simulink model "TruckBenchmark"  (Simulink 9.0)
settings: Solver=ode23s  StartTime=0.0  StopTime=inf  FixedStep=0.1  MaxStep=1  RelTol=1e-3  EnableMultiTasking=on
StartFcn:
  | tic
StopFcn:
  | simt=toc;
  | fprintf('Simulation time %.3f s
  | ',simt)
  | TruckBenchmark_Evaluation
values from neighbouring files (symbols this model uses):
  road = scenario.road    [runSim.m]
undefined symbols (not defined in the file or in its folder): A_egrmax, A_vgtmax, AFs, Area, BSR_opt, C_d, c_egr, c_f1, c_f2, c_fricVec, c_mlin, c_mVec, c_pa, c_pe, c_phi2, c_pi, c_psi2, c_r0, c_r1, c_va, c_vgt1, c_vgt2, c_volVec, c_wphiVec, c_wpsiVec, d_pipe, eta_cmax, eta_igch, eta_sc, eta_tmmax, g, gamma_a, gamma_c, gamma_e, h_tot, J_t, K_t, l_pipe, limit_m_f, limit_n_e, m, model, n_cyl, n_pipe, omega_t_Init, p_amb, p_em_Init, p_im_Init, pi_copt, PI_egropt, Q_c, q_HV, R_a, r_c, R_c, R_e, R_t, rho, scenario, T_1_Init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
libraries: controller x1, simulink x1

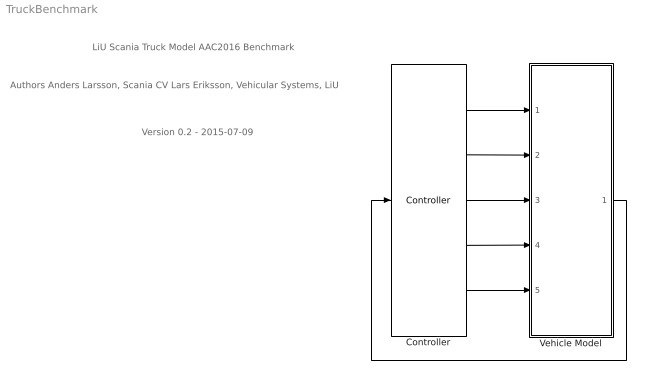
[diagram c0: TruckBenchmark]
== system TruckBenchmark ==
  note: Version 0.2 - 2015-07-09
  note: Authors Anders Larsson, Scania CV Lars Eriksson, Vehicular Systems, LiU
  note: LiU Scania Truck Model AAC2016 Benchmark
  Controller : controller/Controller
  Vehicle Model : Subsystem
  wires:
  Vehicle Model/1(Sensor Buss) -> Controller/1
  Controller/1 -> Vehicle Model/1(gear)
  Controller/2 -> Vehicle Model/2(u_vgt)
  Controller/3 -> Vehicle Model/3(u_egr)
  Controller/4 -> Vehicle Model/4(u_delta)
  Controller/5 -> Vehicle Model/5(F_brake)

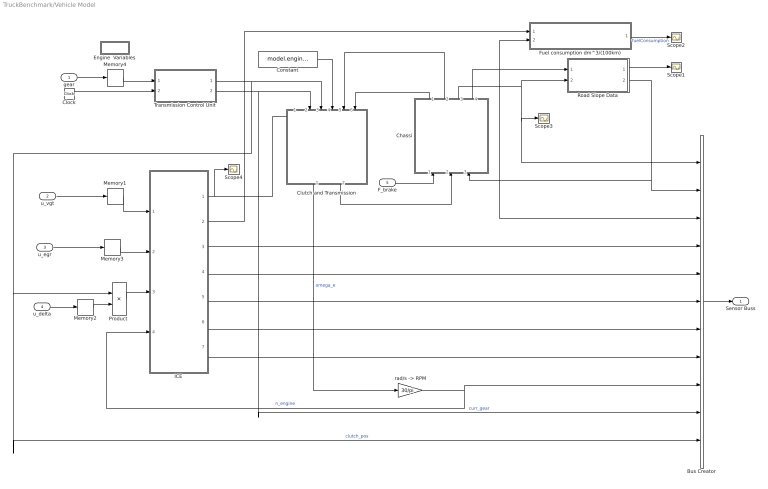
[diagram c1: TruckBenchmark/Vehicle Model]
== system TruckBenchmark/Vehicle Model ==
  gear : Inport
  u_vgt : Inport  Port=2
  u_egr : Inport  Port=3
  u_delta : Inport  Port=4
  F_brake : Inport  Port=5
  Bus Creator : BusCreator  Inputs=11
  Chassi : Subsystem
  Clock : Clock
  Clutch and Transmission : Subsystem
  Constant : Constant  Value=model.engine.J_e
  Engine  Variables : Subsystem
  Fuel consumption dm^3/(100km) : MATLAB Function  TreatAsAtomicUnit=on
  ICE : Subsystem
  Memory1 : Memory  InitialCondition=40
  Memory2 : Memory
  Memory3 : Memory
  Memory4 : Memory  InitialCondition=scenario.gear_init
  "Product " : Product  Inputs=**
  Road Slope Data : Subsystem
  Scope{1..4} (4 alike) : Scope
  Transmission Control Unit : MATLAB Function  TreatAsAtomicUnit=on
  "rad/s -> RPM" : Gain  Gain=30/pi
  Sensor Buss : Outport
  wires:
  ICE/1(M_e) -> Clutch and Transmission/1(M_e [Nm]), Scope4/1
  Road Slope Data/2(slope [rad]) -> Chassi/3(Slope), Bus Creator/2
  Chassi/3(Vehicle Speed[km/h]) -> Road Slope Data/2(v [km/h]), Bus Creator/1, Scope3/1
  ICE/2(m_fuelTot) -> Fuel consumption dm^3/(100km)/1(m_fuelTot)
  Fuel consumption dm^3/(100km)/1(fuelConsumption) -> Scope2/1  "fuelConsumption"
  Chassi/4(Distance [m]) -> Road Slope Data/1(x_distance), Fuel consumption dm^3/(100km)/2(x_distance), Bus Creator/3
  ICE/3(r_lambdaOut) -> Bus Creator/4
  ICE/4(p_inletManifold) -> Bus Creator/5
  ICE/5(r_egr) -> Bus Creator/6
  ICE/6(W_c) -> Bus Creator/7
  u_vgt/1 -> Memory1/1
  u_egr/1 -> Memory3/1
  Memory3/1 -> ICE/2(u_egr)
  F_brake/1 -> Chassi/1(Brake Pedal [%])
  Bus Creator/1 -> Sensor Buss/1
  Clutch and Transmission/2(w_wheel [rad/s]) -> Chassi/2(Wheel speed [rad/s])
  Clutch and Transmission/1(w_e [rad/s]) -> "rad/s -> RPM"/1  "omega_e"
  Chassi/1(Vehicle Inertia [kgm^2]) -> Clutch and Transmission/6(J_veh)
  Chassi/2(Vehicle Torque [Nm]) -> Clutch and Transmission/5(M_veh [Nm])
  "rad/s -> RPM"/1 -> ICE/4(n_e), Bus Creator/9  "n_engine"
  Constant/1 -> Clutch and Transmission/4(J_e)
  Memory1/1 -> ICE/1(u_vgt)
  Transmission Control Unit/2(gear_out) -> Bus Creator/10, Clutch and Transmission/2(Gear)  "curr_gear"
  Clock/1 -> Transmission Control Unit/2(time)
  gear/1 -> Memory4/1
  "Product "/1 -> ICE/3(u_delta)
  Transmission Control Unit/1(clutch) -> Clutch and Transmission/3(Clutch Pos [0...1]), "Product "/1, Bus Creator/11  "clutch_pos"
  u_delta/1 -> Memory2/1
  Memory4/1 -> Transmission Control Unit/1(gear_ref)
  ICE/7(n_t) -> Bus Creator/8
  Road Slope Data/1(altitude [m]) -> Scope1/1
  Memory2/1 -> "Product "/2

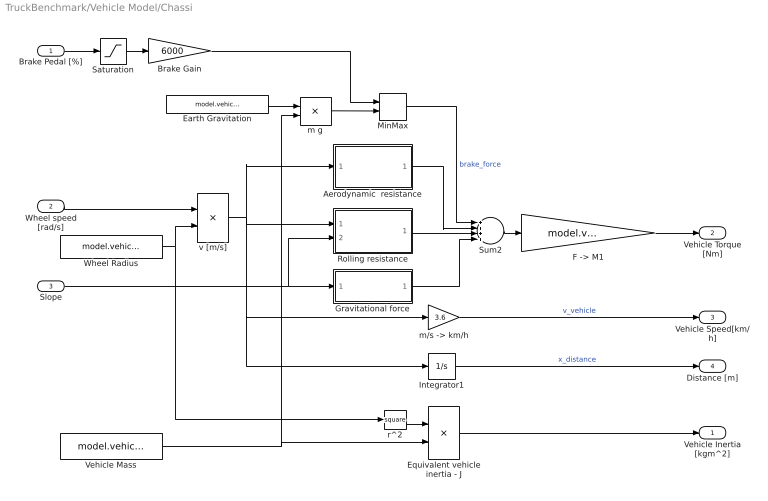
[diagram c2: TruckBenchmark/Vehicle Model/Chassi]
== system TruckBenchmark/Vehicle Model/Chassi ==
  Brake Pedal [%] : Inport
  Wheel speed [rad/s] : Inport  Port=2
  Slope : Inport  Port=3
  Aerodynamic  resistance : Subsystem
  Brake Gain : Gain  Gain=6000
  Earth Gravitation : Constant  Value=model.vehicle.g
  Equivalent vehicle inertia - J : Product
  "F -> M1" : Gain  Gain=model.vehicle.r_w
  Gravitational force : Subsystem
  Integrator1 : Integrator  LimitOutput=on  LowerSaturationLimit=0
  MinMax : MinMax  Inputs=2
  Rolling resistance : Subsystem
  Saturation : Saturate  UpperLimit=100  LowerLimit=0
  Sum2 : Sum  Inputs=++++
  Vehicle Mass : Constant  Value=model.vehicle.m
  Wheel Radius : Constant  Value=model.vehicle.r_w
  m g : Product
  "m/s -> km/h" : Gain  Gain=3.6
  r^2 : Math  Operator=square
  v [m/s] : Product
  Vehicle Inertia [kgm^2] : Outport
  Vehicle Torque [Nm] : Outport  Port=2
  Vehicle Speed[km/h] : Outport  Port=3
  Distance [m] : Outport  Port=4
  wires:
  Brake Pedal [%]/1 -> Saturation/1
  Wheel Radius/1 -> r^2/1, v [m/s]/2
  v [m/s]/1 -> Aerodynamic  resistance/1(v [m/s]), Rolling resistance/1(v [m/s]), Integrator1/1, "m/s -> km/h"/1
  "m/s -> km/h"/1 -> Vehicle Speed[km/h]/1  "v_vehicle"
  "F -> M1"/1 -> Vehicle Torque [Nm]/1
  Equivalent vehicle inertia - J/1 -> Vehicle Inertia [kgm^2]/1
  Wheel speed [rad/s]/1 -> v [m/s]/1
  Sum2/1 -> "F -> M1"/1
  Slope/1 -> Rolling resistance/2(alpha [rad]), Gravitational force/1(alpha [rad])
  r^2/1 -> Equivalent vehicle inertia - J/1
  Vehicle Mass/1 -> m g/2, Equivalent vehicle inertia - J/2
  Integrator1/1 -> Distance [m]/1  "x_distance"
  Brake Gain/1 -> MinMax/1
  m g/1 -> MinMax/2
  Earth Gravitation/1 -> m g/1
  Saturation/1 -> Brake Gain/1
  MinMax/1 -> Sum2/1  "brake_force"
  Aerodynamic  resistance/1(F_a) -> Sum2/2
  Rolling resistance/1(F_r) -> Sum2/3
  Gravitational force/1(F_g) -> Sum2/4

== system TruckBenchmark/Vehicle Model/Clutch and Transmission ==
  M_e [Nm] : Inport
  Gear : Inport  Port=2
  Clutch Pos [0...1] : Inport  Port=3
  J_e : Inport  Port=4
  M_veh [Nm] : Inport  Port=5
  J_veh : Inport  Port=6
  Clutch Transfer : Subsystem
  Engine Dynamics : Subsystem
  Final Drive gear ratio : Gain  Gain=model.transmission.i_f
  Gear box gear ratios : Lookup  InputValues=model.transmission.r_gearNumbers  Table=model.transmission.r_gearRatios
  Mux : Mux  Inputs=5
  Speed Difference Clutch Limits : Subsystem
  Vehicle Dynamics : Subsystem
  w_e [rad/s] : Outport
  w_wheel [rad/s] : Outport  Port=2
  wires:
  M_e [Nm]/1 -> Engine Dynamics/2(Tq_e), Mux/1
  J_e/1 -> Engine Dynamics/3(J_e), Mux/2
  Gear/1 -> Gear box gear ratios/1
  M_veh [Nm]/1 -> Vehicle Dynamics/2(Tq_veh), Mux/3
  J_veh/1 -> Vehicle Dynamics/3(J_v), Mux/4
  Clutch Pos [0...1]/1 -> Speed Difference Clutch Limits/1(Clutch [0...1])
  Engine Dynamics/1(w_e) -> w_e [rad/s]/1, Speed Difference Clutch Limits/2(w_e)  "omega_e"
  Clutch Transfer/1(M_c) -> Vehicle Dynamics/1(Tq_c), Engine Dynamics/1(Tq_c)  "M_c"
  Mux/1 -> Clutch Transfer/3(Insignals)
  Speed Difference Clutch Limits/1(Clutch Locked) -> Clutch Transfer/2(Clutch Locked)  "cl_lock"
  Speed Difference Clutch Limits/2(M_c_max) -> Clutch Transfer/1(Tq_c_max)  "M_c_max"
  Vehicle Dynamics/1(w_wheel) -> w_wheel [rad/s]/1, Speed Difference Clutch Limits/3(w_wheel)  "omega_w"
  Gear box gear ratios/1 -> Final Drive gear ratio/1
  Final Drive gear ratio/1 -> Speed Difference Clutch Limits/4(Gear ratio), Vehicle Dynamics/4(Gear ratio), Mux/5

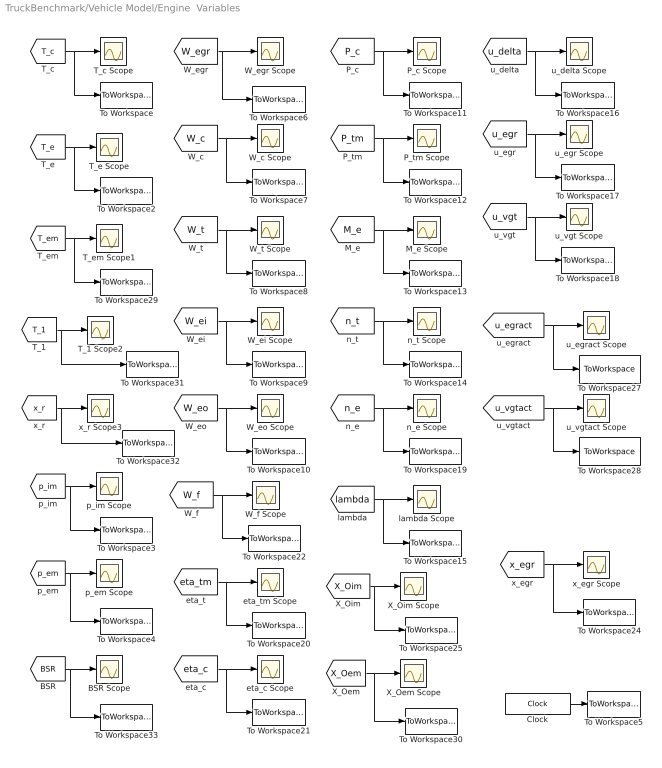
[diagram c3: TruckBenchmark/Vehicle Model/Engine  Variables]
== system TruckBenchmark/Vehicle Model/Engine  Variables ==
  BSR Scope : Scope
  Clock : Clock
  M_e Scope : Scope
  P_c Scope : Scope
  P_tm Scope : Scope
  T_1 Scope2 : Scope
  T_c Scope : Scope
  T_e Scope : Scope
  T_em Scope1 : Scope
  To Workspace : ToWorkspace  VariableName=simT_c  SampleTime=-1
  To Workspace10 : ToWorkspace  VariableName=simW_eo  SampleTime=-1
  To Workspace11 : ToWorkspace  VariableName=simP_c  SampleTime=-1
  To Workspace12 : ToWorkspace  VariableName=simP_tm  SampleTime=-1
  To Workspace13 : ToWorkspace  VariableName=simM_e  SampleTime=-1
  To Workspace14 : ToWorkspace  VariableName=simn_t  SampleTime=-1
  To Workspace15 : ToWorkspace  VariableName=simlambda  SampleTime=-1
  To Workspace16 : ToWorkspace  VariableName=simu_delta  SampleTime=-1
  To Workspace17 : ToWorkspace  VariableName=simu_egr  SampleTime=-1
  To Workspace18 : ToWorkspace  VariableName=simu_vgt  SampleTime=-1
  To Workspace19 : ToWorkspace  VariableName=simn_e  SampleTime=-1
  To Workspace2 : ToWorkspace  VariableName=simT_e  SampleTime=-1
  To Workspace20 : ToWorkspace  VariableName=simeta_tm  SampleTime=-1
  To Workspace21 : ToWorkspace  VariableName=simeta_c  SampleTime=-1
  To Workspace22 : ToWorkspace  VariableName=simW_f  SampleTime=-1
  To Workspace24 : ToWorkspace  VariableName=simx_egr  SampleTime=-1
  To Workspace25 : ToWorkspace  VariableName=simX_Oim  SampleTime=-1
  To Workspace27 : ToWorkspace  VariableName=simu_egract  SampleTime=-1
  To Workspace28 : ToWorkspace  VariableName=simu_vgtact  SampleTime=-1
  To Workspace29 : ToWorkspace  VariableName=simT_em  SampleTime=-1
  To Workspace3 : ToWorkspace  VariableName=simp_im  SampleTime=-1
  To Workspace30 : ToWorkspace  VariableName=simX_Oem  SampleTime=-1
  To Workspace31 : ToWorkspace  VariableName=simT_1  SampleTime=-1
  To Workspace32 : ToWorkspace  VariableName=simx_r  SampleTime=-1
  To Workspace33 : ToWorkspace  VariableName=simBSR  SampleTime=-1
  To Workspace4 : ToWorkspace  VariableName=simp_em  SampleTime=-1
  To Workspace5 : ToWorkspace  VariableName=simTime  SampleTime=-1
  To Workspace6 : ToWorkspace  VariableName=simW_egr  SampleTime=-1
  To Workspace7 : ToWorkspace  VariableName=simW_c  SampleTime=-1
  To Workspace8 : ToWorkspace  VariableName=simW_t  SampleTime=-1
  To Workspace9 : ToWorkspace  VariableName=simW_ei  SampleTime=-1
  W_c Scope : Scope
  W_egr Scope : Scope
  W_ei Scope : Scope
  W_eo Scope : Scope
  W_f Scope : Scope
  W_t Scope : Scope
  X_Oem Scope : Scope
  X_Oim Scope : Scope
  eta_c Scope : Scope
  eta_tm Scope : Scope
  lambda Scope : Scope
  n_e Scope : Scope
  n_t Scope : Scope
  p_em Scope : Scope
  p_im Scope : Scope
  u_delta Scope : Scope
  u_egr Scope : Scope
  u_egract Scope : Scope
  u_vgt Scope : Scope
  u_vgtact Scope : Scope
  x_egr Scope : Scope
  x_r Scope3 : Scope
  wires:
  [u_vgtact] -> To Workspace28/1, u_vgtact Scope/1
  [u_egract] -> u_egract Scope/1, To Workspace27/1
  [x_egr] -> x_egr Scope/1, To Workspace24/1
  [W_f] -> W_f Scope/1, To Workspace22/1
  [eta_c] -> To Workspace21/1, eta_c Scope/1
  [eta_tm] -> eta_tm Scope/1, To Workspace20/1
  [n_e] -> n_e Scope/1, To Workspace19/1
  [u_vgt] -> u_vgt Scope/1, To Workspace18/1
  [u_egr] -> To Workspace17/1, u_egr Scope/1
  [u_delta] -> u_delta Scope/1, To Workspace16/1
  Clock/1 -> To Workspace5/1
  [lambda] -> To Workspace15/1, lambda Scope/1
  [M_e] -> To Workspace13/1, M_e Scope/1
  [W_eo] -> To Workspace10/1, W_eo Scope/1
  [P_tm] -> To Workspace12/1, P_tm Scope/1
  [P_c] -> To Workspace11/1, P_c Scope/1
  [W_ei] -> To Workspace9/1, W_ei Scope/1
  [W_t] -> To Workspace8/1, W_t Scope/1
  [W_c] -> To Workspace7/1, W_c Scope/1
  [W_egr] -> To Workspace6/1, W_egr Scope/1
  [n_t] -> To Workspace14/1, n_t Scope/1
  [p_em] -> To Workspace4/1, p_em Scope/1
  [p_im] -> To Workspace3/1, p_im Scope/1
  [T_e] -> To Workspace2/1, T_e Scope/1
  [T_c] -> To Workspace/1, T_c Scope/1
  [T_em] -> T_em Scope1/1, To Workspace29/1
  [X_Oem] -> X_Oem Scope/1, To Workspace30/1
  [X_Oim] -> X_Oim Scope/1, To Workspace25/1
  [T_1] -> T_1 Scope2/1, To Workspace31/1
  [x_r] -> x_r Scope3/1, To Workspace32/1
  [BSR] -> BSR Scope/1, To Workspace33/1

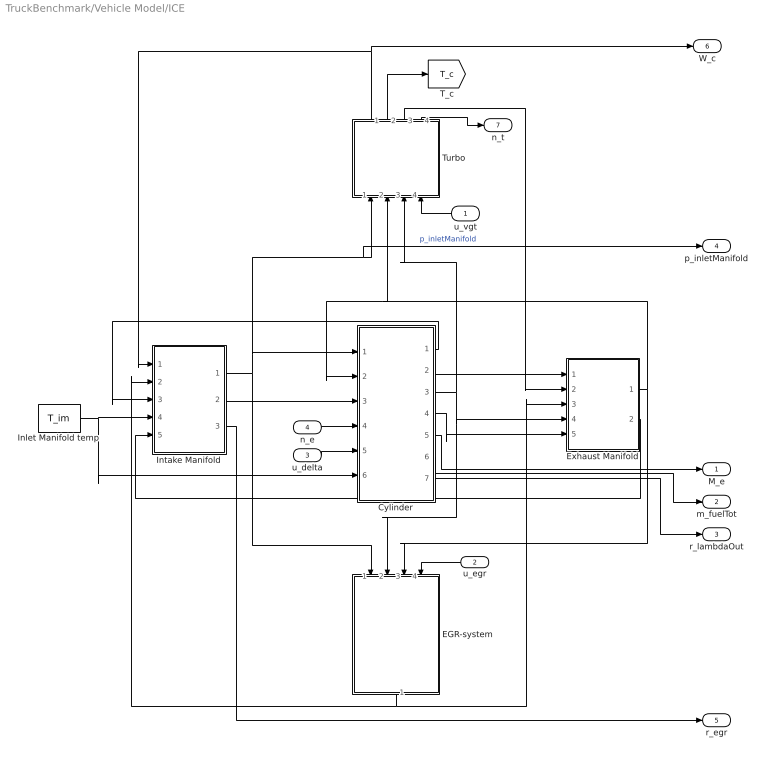
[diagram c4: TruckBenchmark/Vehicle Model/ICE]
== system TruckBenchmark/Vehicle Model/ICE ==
  u_vgt : Inport
  u_egr : Inport  Port=2
  u_delta : Inport  Port=3
  n_e : Inport  Port=4
  Cylinder : Subsystem
  EGR-system : Subsystem
  Exhaust Manifold : Subsystem
  Inlet Manifold temp : Constant  Value=T_im
  Intake Manifold : Subsystem
  Turbo : Subsystem
  M_e : Outport
  m_fuelTot : Outport  Port=2
  r_lambdaOut : Outport  Port=3
  p_inletManifold : Outport  Port=4
  r_egr : Outport  Port=5
  W_c : Outport  Port=6
  n_t : Outport  Port=7
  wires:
  Exhaust Manifold/2(X_Oem) -> Intake Manifold/5(X_Oem)
  Cylinder/4(X_Oe) -> Exhaust Manifold/5(X_Oe)
  Intake Manifold/2(X_Oim) -> Cylinder/3(X_Oim)
  u_delta/1 -> Cylinder/5(u_delta)
  n_e/1 -> Cylinder/4(n_e)
  Turbo/2(T_c) -> [T_c]
  u_vgt/1 -> Turbo/4(u_vgt)
  u_egr/1 -> EGR-system/4(u_egr)
  Cylinder/3(T_em) -> EGR-system/2(T_em), Exhaust Manifold/4(T_em), Turbo/3(T_em)
  Cylinder/1(W_ei) -> Intake Manifold/3(W_ei)
  Inlet Manifold temp/1 -> Intake Manifold/4(T_im), Cylinder/6(T_im)
  Turbo/1(W_c) -> Intake Manifold/1(W_c), W_c/1
  EGR-system/1(W_egr) -> Intake Manifold/2(W_egr), Exhaust Manifold/3(W_egr)
  Turbo/3(W_t) -> Exhaust Manifold/2(W_t)
  Cylinder/2(W_eo) -> Exhaust Manifold/1(W_eo)
  Exhaust Manifold/1(p_em) -> EGR-system/3(p_em), Cylinder/2(p_em), Turbo/2(p_em)
  Intake Manifold/1(p_im) -> p_inletManifold/1, Turbo/1(p_im), Cylinder/1(p_im), EGR-system/1(p_im)  "p_inletManifold"
  Cylinder/5(M_e) -> M_e/1
  Cylinder/6(m_fuelTot) -> m_fuelTot/1
  Cylinder/7(r_lambdaOut) -> r_lambdaOut/1
  Intake Manifold/3(r_egr) -> r_egr/1
  Turbo/4(n_t) -> n_t/1

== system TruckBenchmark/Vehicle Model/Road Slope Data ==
  x_distance : Inport
  v [km/h] : Inport  Port=2
  1-D Lookup Table : Lookup_n-D  NumberOfTableDimensions=1  BreakpointsForDimension1=road.x_distanceVector  BeginIndexSearchUsingPreviousIndexResult=on  Table=road.k_slopeVector  InterpMethod=Cubic spline  RndMeth=Simplest
  Constant : Constant  Value=road.x_distanceVector(end)
  Integrator : Integrator  InitialCondition=scenario.h_0  LowerSaturationLimit=0
  Relational Operator : RelationalOperator  OutDataTypeStr=boolean
  Scope1 : Scope
  Scope2 : Scope
  Stop Simulation : Stop
  Trigonometric Function : Trigonometry
  h dot : Product  Inputs=**
  "km/h -> m/s " : Gain  Gain=1/3.6
  altitude [m] : Outport
  slope [rad] : Outport  Port=2
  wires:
  x_distance/1 -> Relational Operator/1, 1-D Lookup Table/1, Scope2/1
  1-D Lookup Table/1 -> Trigonometric Function/1, slope [rad]/1, Scope1/1  "k_slope"
  Constant/1 -> Relational Operator/2
  Relational Operator/1 -> Stop Simulation/1
  v [km/h]/1 -> "km/h -> m/s "/1
  Trigonometric Function/1 -> h dot/1
  "km/h -> m/s "/1 -> h dot/2
  h dot/1 -> Integrator/1
  Integrator/1 -> altitude [m]/1  "altitude"

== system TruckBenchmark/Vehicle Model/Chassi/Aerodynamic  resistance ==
  v [m/s] : Inport
  0.5*rho_air*A*C_d : Gain  Gain=0.5*rho*C_d*Area
  v^2 : Math  Operator=square
  F_a : Outport
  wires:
  v [m/s]/1 -> v^2/1
  v^2/1 -> 0.5*rho_air*A*C_d/1
  0.5*rho_air*A*C_d/1 -> F_a/1  "F_a"

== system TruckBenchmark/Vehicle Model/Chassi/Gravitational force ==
  alpha [rad] : Inport
  Trigonometric Function : Trigonometry
  m g : Constant  Value=m*g
  mult2 : Product
  F_g : Outport
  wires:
  alpha [rad]/1 -> Trigonometric Function/1
  m g/1 -> mult2/2
  mult2/1 -> F_g/1  "F_g"
  Trigonometric Function/1 -> mult2/1

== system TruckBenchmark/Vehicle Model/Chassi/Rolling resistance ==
  v [m/s] : Inport
  alpha [rad] : Inport  Port=2
  Math Function : Math  Operator=square
  Sum1 : Sum
  Trigonometric Function : Trigonometry  Operator=cos
  c_r0 : Constant  Value=c_r0
  c_r1 : Constant  Value=c_r1
  const : Constant  Value=3.6
  m g : Constant  Value=m*g
  mult{,1..3} (4 alike) : Product
  F_r : Outport
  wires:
  v [m/s]/1 -> mult3/1
  Sum1/1 -> mult1/1
  mult1/1 -> F_r/1  "F_r"
  c_r0/1 -> Sum1/2
  mult/1 -> Sum1/1
  c_r1/1 -> mult/2
  m g/1 -> mult2/2
  alpha [rad]/1 -> Trigonometric Function/1
  mult2/1 -> mult1/2
  Trigonometric Function/1 -> mult2/1
  const/1 -> mult3/2
  mult3/1 -> Math Function/1  "v [km/h]"
  Math Function/1 -> mult/1

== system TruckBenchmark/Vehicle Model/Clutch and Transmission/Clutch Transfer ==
  Tq_c_max : Inport
  Clutch Locked : Inport  Port=2
  Insignals : Inport  Port=3
  Abs : Abs
  Abs1 : Abs
  Calc Mc : Fcn  Expr=(u(1)*u(4)/(u(5)^2) + u(2)*u(3)/u(5)) / (u(2) + u(4)/(u(5)^2))
  Logical Operator : Logic  AllPortsSameDT=off  OutDataTypeStr=boolean
  Relational Operator : RelationalOperator  Operator=<  OutDataTypeStr=boolean
  Switch : Switch  Threshold=0.5
  M_c : Outport
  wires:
  Switch/1 -> M_c/1
  Calc Mc/1 -> Abs/1, Switch/1
  Insignals/1 -> Calc Mc/1
  Tq_c_max/1 -> Abs1/1, Switch/3
  Logical Operator/1 -> Switch/2
  Clutch Locked/1 -> Logical Operator/1
  Abs/1 -> Relational Operator/1
  Abs1/1 -> Relational Operator/2
  Relational Operator/1 -> Logical Operator/2

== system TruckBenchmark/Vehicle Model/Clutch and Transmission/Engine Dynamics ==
  Tq_c : Inport
  Tq_e : Inport  Port=2
  J_e : Inport  Port=3
  Integrator1 : Integrator  InitialCondition=600*pi/30  LimitOutput=on  LowerSaturationLimit=450*pi/30
  Sum2 : Sum  Inputs=-+|
  w dot4 : Product  Inputs=*/
  w_e : Outport
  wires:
  w dot4/1 -> Integrator1/1
  Sum2/1 -> w dot4/1
  J_e/1 -> w dot4/2
  Integrator1/1 -> w_e/1
  Tq_c/1 -> Sum2/1
  Tq_e/1 -> Sum2/2

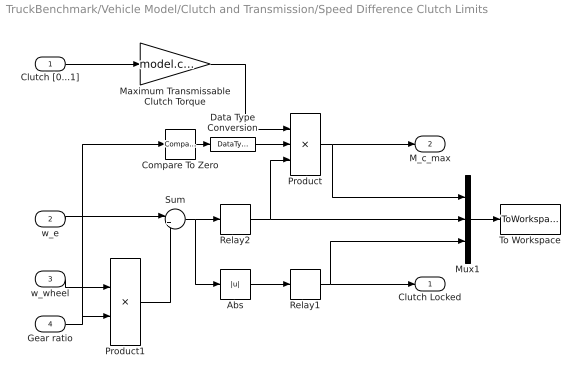
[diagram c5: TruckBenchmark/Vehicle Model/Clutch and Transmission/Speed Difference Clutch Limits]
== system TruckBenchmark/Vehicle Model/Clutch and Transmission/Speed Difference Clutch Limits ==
  Clutch [0...1] : Inport
  w_e : Inport  Port=2
  w_wheel : Inport  Port=3
  Gear ratio : Inport  Port=4
  Abs : Abs
  Compare To Zero : simulink/Logic and Bit Operations/Compare To Zero  relop=>  OutDataTypeStr=uint8
  Data Type Conversion : DataTypeConversion
  Maximum Transmissable Clutch Torque : Gain  Gain=model.clutch.M_max
  Mux1 : Mux  Inputs=3
  Product : Product  Inputs=3
  Product1 : Product
  Relay1 : Relay  OnSwitchValue=1  OffSwitchValue=1e-1  OnOutputValue=0  OffOutputValue=1
  Relay2 : Relay  OnSwitchValue=1e-1  OffSwitchValue=-1e-1  OffOutputValue=-1
  Sum : Sum  Inputs=|+-
  To Workspace : ToWorkspace  VariableName=C  SaveFormat=Structure With Time  SampleTime=-1
  Clutch Locked : Outport
  M_c_max : Outport  Port=2
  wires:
  Relay2/1 -> Product/3, Mux1/2
  Abs/1 -> Relay1/1
  Sum/1 -> Relay2/1, Abs/1
  Clutch [0...1]/1 -> Maximum Transmissable Clutch Torque/1
  w_e/1 -> Sum/1
  Gear ratio/1 -> Compare To Zero/1, Product1/2
  w_wheel/1 -> Product1/1
  Maximum Transmissable Clutch Torque/1 -> Product/1
  Relay1/1 -> Clutch Locked/1, Mux1/3
  Mux1/1 -> To Workspace/1
  Product/1 -> Mux1/1, M_c_max/1
  Product1/1 -> Sum/2
  Compare To Zero/1 -> Data Type Conversion/1
  Data Type Conversion/1 -> Product/2

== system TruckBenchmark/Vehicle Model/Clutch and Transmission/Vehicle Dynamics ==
  Tq_c : Inport
  Tq_veh : Inport  Port=2
  J_v : Inport  Port=3
  Gear ratio : Inport  Port=4
  Integrator : Integrator  LimitOutput=on  LowerSaturationLimit=0
  Sum1 : Sum  Inputs=|+-
  w dot3 : Product  Inputs=**
  w dot5 : Product  Inputs=*/
  w_wheel : Outport
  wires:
  Gear ratio/1 -> w dot3/2
  J_v/1 -> w dot5/2
  Tq_c/1 -> w dot3/1
  Tq_veh/1 -> Sum1/2
  w dot3/1 -> Sum1/1
  Sum1/1 -> w dot5/1
  w dot5/1 -> Integrator/1
  Integrator/1 -> w_wheel/1

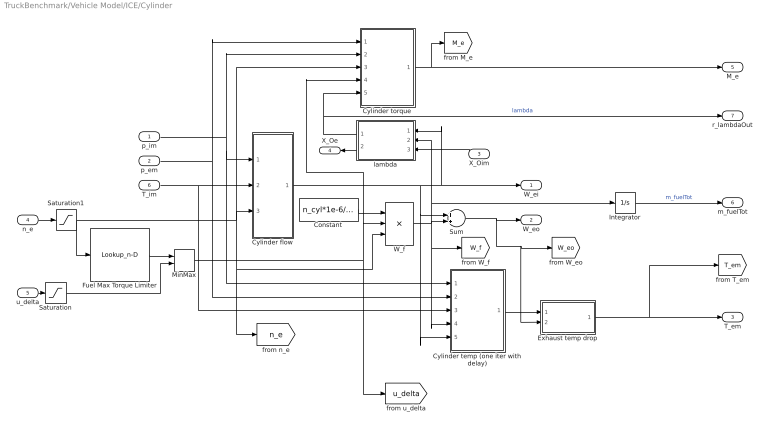
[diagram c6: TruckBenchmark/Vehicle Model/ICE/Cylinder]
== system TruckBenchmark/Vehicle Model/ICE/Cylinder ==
  p_im : Inport
  p_em : Inport  Port=2
  X_Oim : Inport  Port=3
  n_e : Inport  Port=4
  u_delta : Inport  Port=5
  T_im : Inport  Port=6
  Constant : Constant  Value=n_cyl*1e-6/120
  Cylinder flow : Subsystem
  Cylinder temp (one iter with delay) : Subsystem
  Cylinder torque : Subsystem
  Exhaust temp drop : Subsystem
  Fuel Max Torque Limiter : Lookup_n-D  NumberOfTableDimensions=1  BreakpointsForDimension1=limit_n_e  Table=limit_m_f  RndMeth=Simplest
  Integrator : Integrator
  MinMax : MinMax  Inputs=2
  Saturation : Saturate  UpperLimit=340  LowerLimit=0
  Saturation1 : Saturate  UpperLimit=2000  LowerLimit=400
  Sum : Sum
  W_f : Product  Inputs=3
  lambda : Subsystem
  W_ei : Outport
  W_eo : Outport  Port=2
  T_em : Outport  Port=3
  X_Oe : Outport  Port=4
  M_e : Outport  Port=5
  m_fuelTot : Outport  Port=6
  r_lambdaOut : Outport  Port=7
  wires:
  lambda/2(X_Oe) -> X_Oe/1
  n_e/1 -> Saturation1/1
  X_Oim/1 -> lambda/3(X_Oim)
  lambda/1(lambda_out) -> r_lambdaOut/1, Cylinder torque/5(lambda)  "lambda"
  Cylinder temp (one iter with delay)/1(T_e) -> Exhaust temp drop/1(T_in)
  Cylinder torque/1(M_e) -> [M_e], M_e/1
  u_delta/1 -> Saturation/1
  Constant/1 -> W_f/1
  W_f/1 -> Integrator/1, lambda/2(W_f), [W_f], Cylinder temp (one iter with delay)/4(W_f), Sum/2
  Sum/1 -> Exhaust temp drop/2(W), [W_eo], W_eo/1
  Cylinder flow/1(W_ei) -> lambda/1(W_ei), W_ei/1, Cylinder temp (one iter with delay)/5(W_ei), Sum/1
  T_im/1 -> Cylinder temp (one iter with delay)/3(T_im), Cylinder flow/2(T_im)
  p_em/1 -> Cylinder temp (one iter with delay)/2(p_em), Cylinder torque/1(p_em)
  p_im/1 -> Cylinder temp (one iter with delay)/1(p_im), Cylinder flow/1(p_im), Cylinder torque/2(p_im)
  Exhaust temp drop/1(T_out) -> [T_em], T_em/1
  Saturation1/1 -> Fuel Max Torque Limiter/1, Cylinder flow/3(n_e), [n_e], W_f/3, Cylinder torque/3(n_e)
  Integrator/1 -> m_fuelTot/1  "m_fuelTot"
  Saturation/1 -> MinMax/2
  Fuel Max Torque Limiter/1 -> MinMax/1
  MinMax/1 -> Cylinder torque/4(u_delta), W_f/2, [u_delta]

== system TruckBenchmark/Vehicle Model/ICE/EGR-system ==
  p_im : Inport
  T_em : Inport  Port=2
  p_em : Inport  Port=3
  u_egr : Inport  Port=4
  Constant : Constant  Value=model.engine.with_egr_act_model
  EGR act : Subsystem
  Fcn W_egr : Fcn  Expr=A_egrmax*u[1]*u[3]*u[2]/sqrt(u[4]*R_e)
  Mux : Mux
  PI_egr : Product  Inputs=*/
  PSI_egr : Subsystem
  Saturation : Saturate  UpperLimit=100  LowerLimit=0
  Switch : Switch  Threshold=0.5
  f_egr : Subsystem
  W_egr : Outport
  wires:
  Constant/1 -> Switch/2
  EGR act/1(Out) -> Switch/1
  Switch/1 -> [u_egract], f_egr/1(u_egr)
  u_egr/1 -> Saturation/1
  Fcn W_egr/1 -> [W_egr], W_egr/1
  T_em/1 -> Mux/4
  PSI_egr/1(PSI_egr) -> Mux/2
  f_egr/1(f_egr) -> Mux/1
  Mux/1 -> Fcn W_egr/1
  PI_egr/1 -> PSI_egr/1(PI_egr)
  p_em/1 -> Mux/3, PI_egr/2
  p_im/1 -> PI_egr/1
  Saturation/1 -> EGR act/1(In), Switch/3, [u_egr]

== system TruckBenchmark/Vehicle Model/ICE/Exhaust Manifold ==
  W_eo : Inport
  W_t : Inport  Port=2
  W_egr : Inport  Port=3
  T_em : Inport  Port=4
  X_Oe : Inport  Port=5
  Fcn : Fcn  Expr=R_e*u[1]*u[2]/V_em
  Integrator p_em : Integrator  InitialCondition=p_em_Init  LimitOutput=on  UpperSaturationLimit=20*p_amb  LowerSaturationLimit=0.5*p_amb
  Mux : Mux  Inputs=2
  Subsystem : Subsystem
  Sum : Sum  Inputs=+--
  p_em : Outport
  X_Oem : Outport  Port=2
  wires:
  Subsystem/1(X_Oem) -> [X_Oem], X_Oem/1
  X_Oe/1 -> Subsystem/4(X_Oe)
  Integrator p_em/1 -> Subsystem/1(p_em), [p_em], p_em/1
  W_eo/1 -> Subsystem/3(W_eo), Sum/1
  W_t/1 -> Sum/2
  W_egr/1 -> Sum/3
  Sum/1 -> Mux/1
  T_em/1 -> Subsystem/2(T_em), Mux/2
  Mux/1 -> Fcn/1
  Fcn/1 -> Integrator p_em/1

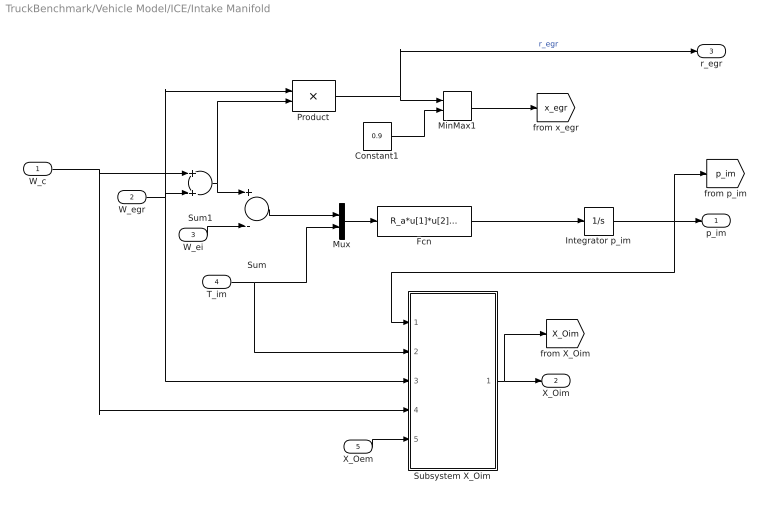
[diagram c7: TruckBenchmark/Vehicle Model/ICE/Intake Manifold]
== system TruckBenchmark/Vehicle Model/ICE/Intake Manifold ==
  W_c : Inport
  W_egr : Inport  Port=2
  W_ei : Inport  Port=3
  T_im : Inport  Port=4
  X_Oem : Inport  Port=5
  Constant1 : Constant  Value=0.9
  Fcn : Fcn  Expr=R_a*u[1]*u[2]/V_im
  Integrator p_im : Integrator  InitialCondition=p_im_Init  LimitOutput=on  UpperSaturationLimit=10*p_amb  LowerSaturationLimit=0.5*p_amb
  MinMax1 : MinMax  Inputs=2
  Mux : Mux  Inputs=2
  Product : Product  Inputs=*/
  Subsystem X_Oim : Subsystem
  Sum : Sum  Inputs=+-
  Sum1 : Sum
  p_im : Outport
  X_Oim : Outport  Port=2
  r_egr : Outport  Port=3
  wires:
  Subsystem X_Oim/1(X_Oim) -> [X_Oim], X_Oim/1
  X_Oem/1 -> Subsystem X_Oim/5(X_Oem)
  Product/1 -> r_egr/1, MinMax1/1  "r_egr"
  Constant1/1 -> MinMax1/2
  W_egr/1 -> Subsystem X_Oim/3(W_egr), Product/1, Sum1/2
  W_c/1 -> Subsystem X_Oim/4(W_c), Sum1/1
  Sum1/1 -> Product/2, Sum/1
  Fcn/1 -> Integrator p_im/1
  Mux/1 -> Fcn/1
  T_im/1 -> Subsystem X_Oim/2(T_im), Mux/2
  Sum/1 -> Mux/1
  W_ei/1 -> Sum/2
  Integrator p_im/1 -> Subsystem X_Oim/1(p_im), [p_im], p_im/1
  MinMax1/1 -> [x_egr]

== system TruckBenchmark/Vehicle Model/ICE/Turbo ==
  p_im : Inport
  p_em : Inport  Port=2
  T_em : Inport  Port=3
  u_vgt : Inport  Port=4
  Compressor : Subsystem
  Turbine : Subsystem
  Turbo inertia : Subsystem
  amb pres : Constant  Value=p_amb
  amb temp : Constant  Value=T_amb
  "rad/s -> RPM" : Gain  Gain=30/pi
  W_c : Outport
  T_c : Outport  Port=2
  W_t : Outport  Port=3
  n_t : Outport  Port=4
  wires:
  u_vgt/1 -> Turbine/5(u_vgt)
  T_em/1 -> Turbine/1(T_em)
  p_em/1 -> Turbine/2(p_em)
  Turbine/1(W_t) -> W_t/1
  Compressor/2(T_c) -> T_c/1
  Compressor/1(W_c) -> W_c/1
  Compressor/3(P_c) -> Turbo inertia/2(P_c)
  Turbine/2(P_t*eta_m) -> Turbo inertia/1(P_t*eta_m)
  Turbo inertia/1(omega_t) -> Turbine/4(omega_t), "rad/s -> RPM"/1, Compressor/4(omega_t)
  p_im/1 -> Compressor/3(p_c)
  amb pres/1 -> Turbine/3(p_es), Compressor/2(p_bc)
  amb temp/1 -> Compressor/1(T_bc)
  "rad/s -> RPM"/1 -> n_t/1  "n_t"

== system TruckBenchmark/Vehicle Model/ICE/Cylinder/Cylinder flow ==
  p_im : Inport
  T_im : Inport  Port=2
  n_e : Inport  Port=3
  Constant : Constant  Value=V_d/(R_a*60*2)
  Mux : Mux  Inputs=2
  Product W_ei : Product  Inputs=***/*
  n_vol : Fcn  Expr=c_volVec(1)*sqrt(u[1])+c_volVec(2)*sqrt(u[2])+c_volVec(3)
  W_ei : Outport
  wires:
  Mux/1 -> n_vol/1
  Product W_ei/1 -> [W_ei], W_ei/1
  Constant/1 -> Product W_ei/5
  T_im/1 -> Product W_ei/4
  n_e/1 -> Mux/2, Product W_ei/3
  n_vol/1 -> Product W_ei/1
  p_im/1 -> Mux/1, Product W_ei/2

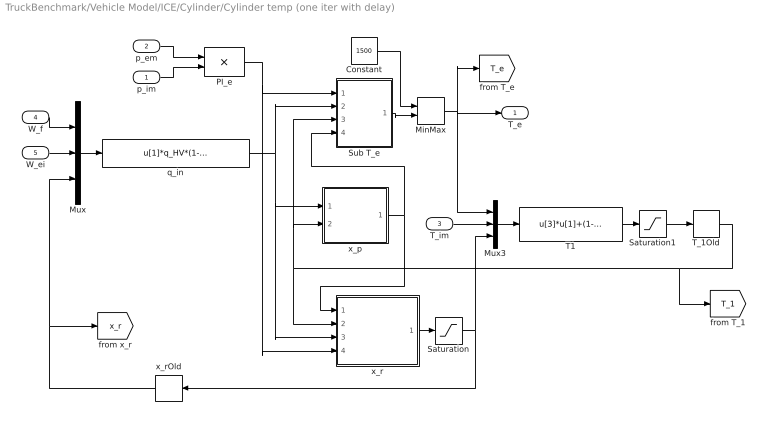
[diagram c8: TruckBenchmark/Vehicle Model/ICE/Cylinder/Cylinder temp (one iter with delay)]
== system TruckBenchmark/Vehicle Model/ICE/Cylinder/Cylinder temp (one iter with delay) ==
  p_im : Inport
  p_em : Inport  Port=2
  T_im : Inport  Port=3
  W_f : Inport  Port=4
  W_ei : Inport  Port=5
  Constant : Constant  Value=1500
  MinMax : MinMax  Inputs=2
  Mux : Mux  Inputs=3
  Mux3 : Mux  Inputs=3
  PI_e : Product  Inputs=*/
  Saturation : Saturate  UpperLimit=1  LowerLimit=0
  Saturation1 : Saturate  UpperLimit=inf  LowerLimit=273
  Sub T_e : Subsystem
  T1 : Fcn  Expr=u[3]*u[1]+(1-u[3])*u[2]
  T_1Old : Memory  InitialCondition=T_1_Init  InheritSampleTime=on
  q_in : Fcn  Expr=u[1]*q_HV*(1-u[3])/(u[1]+u[2])
  x_p : Subsystem
  x_r : Subsystem
  x_rOld : Memory  InitialCondition=x_r_Init  InheritSampleTime=on
  T_e : Outport
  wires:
  Saturation1/1 -> T_1Old/1
  Saturation/1 -> x_rOld/1, Mux3/3
  Constant/1 -> MinMax/1
  Sub T_e/1(T_e) -> MinMax/2
  MinMax/1 -> [T_e], Mux3/1, T_e/1
  x_rOld/1 -> Mux/3, [x_r]
  x_r/1(x_r) -> Saturation/1
  T_1Old/1 -> [T_1], x_r/2(T1), x_p/2(T1), Sub T_e/3(T1)
  T1/1 -> Saturation1/1
  T_im/1 -> Mux3/2
  Mux3/1 -> T1/1
  x_p/1(x_p) -> x_r/1(x_p), Sub T_e/4(x_p)
  PI_e/1 -> x_r/4(PI_e), Sub T_e/1(PI_e)
  q_in/1 -> Sub T_e/2(q_in), x_p/1(q_in), x_r/3(q_in)
  W_ei/1 -> Mux/2
  W_f/1 -> Mux/1
  Mux/1 -> q_in/1
  p_em/1 -> PI_e/1
  p_im/1 -> PI_e/2

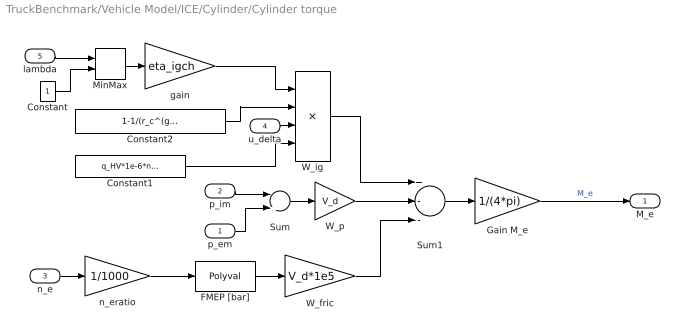
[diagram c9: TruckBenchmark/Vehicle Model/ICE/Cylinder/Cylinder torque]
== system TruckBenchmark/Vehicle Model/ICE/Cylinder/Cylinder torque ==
  p_em : Inport
  p_im : Inport  Port=2
  n_e : Inport  Port=3
  u_delta : Inport  Port=4
  lambda : Inport  Port=5
  Constant : Constant
  Constant1 : Constant  Value=q_HV*1e-6*n_cyl
  Constant2 : Constant  Value=1-1/(r_c^(gamma_c-1))
  FMEP [bar] : Polyval  Coefs=c_fricVec
  Gain M_e : Gain  Gain=1/(4*pi)
  MinMax : MinMax  Inputs=2
  Sum : Sum  Inputs=-+
  Sum1 : Sum  Inputs=+--
  W_fric : Gain  Gain=V_d*1e5
  W_ig : Product  Inputs=4
  W_p : Gain  Gain=V_d
  gain : Gain  Gain=eta_igch
  n_eratio : Gain  Gain=1/1000
  M_e : Outport
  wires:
  Gain M_e/1 -> M_e/1  "M_e"
  Constant1/1 -> W_ig/4
  u_delta/1 -> W_ig/3
  Constant2/1 -> W_ig/2
  Sum1/1 -> Gain M_e/1
  W_fric/1 -> Sum1/3
  W_p/1 -> Sum1/2
  W_ig/1 -> Sum1/1
  FMEP [bar]/1 -> W_fric/1
  n_eratio/1 -> FMEP [bar]/1
  n_e/1 -> n_eratio/1
  gain/1 -> W_ig/1
  MinMax/1 -> gain/1
  Constant/1 -> MinMax/2
  lambda/1 -> MinMax/1
  Sum/1 -> W_p/1
  p_em/1 -> Sum/2
  p_im/1 -> Sum/1

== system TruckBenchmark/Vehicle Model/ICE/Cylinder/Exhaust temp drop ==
  T_in : Inport
  W : Inport  Port=2
  Fcn T_out : Fcn  Expr=T_w+(u[1]-T_w)*exp(-1*h_tot*pi*d_pipe*l_pipe*n_pipe/(u[2]*c_pe))
  Mux : Mux  Inputs=2
  T_out : Outport
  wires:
  Fcn T_out/1 -> T_out/1
  Mux/1 -> Fcn T_out/1
  W/1 -> Mux/2
  T_in/1 -> Mux/1

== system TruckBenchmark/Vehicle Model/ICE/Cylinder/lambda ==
  note: Avoid division by Zero
  W_ei : Inport
  W_f : Inport  Port=2
  X_Oim : Inport  Port=3
  Constant1 : Constant  Value=AFs*X_Oc
  Constant2 : Constant  Value=0
  Fcn : Fcn  Expr=(u[1]*u[3]-u[2]*AFs*X_Oc)/(u[1]+u[2])
  Fuel Limit : Constant  Value=1e-5
  Max1 : MinMax  Function=max  Inputs=2
  MinMax : MinMax  Function=max  Inputs=2
  Mux : Mux  Inputs=3
  lambda : Product  Inputs=/*/*
  lambda_out : Outport
  X_Oe : Outport  Port=2
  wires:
  Constant2/1 -> MinMax/2
  Fcn/1 -> MinMax/1
  MinMax/1 -> X_Oe/1
  Mux/1 -> Fcn/1
  X_Oim/1 -> Mux/3, lambda/4
  Max1/1 -> Mux/2, lambda/3
  W_ei/1 -> Mux/1, lambda/2
  lambda/1 -> lambda_out/1, [lambda]  "r_lambdaOut"
  Constant1/1 -> lambda/1
  Fuel Limit/1 -> Max1/2
  W_f/1 -> Max1/1

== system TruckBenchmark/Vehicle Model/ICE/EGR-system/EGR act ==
  In : Inport
  Actuator1 : Subsystem
  Actuator2 : Subsystem
  Gain : Gain  Gain=model.engine.K_egr
  Gain1 : Gain  Gain=model.engine.K_egr-1
  Subtract : Sum  Inputs=+-
  Transport Delay : TransportDelay  DelayTime=model.engine.tau_degr  InitialOutput=model.engine.uInit_egr
  Out : Outport
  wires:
  Gain1/1 -> Subtract/2
  Gain/1 -> Subtract/1
  Actuator2/1(Out) -> Gain1/1
  Actuator1/1(Out) -> Gain/1
  Transport Delay/1 -> Actuator2/1(In), Actuator1/1(In)
  Subtract/1 -> Out/1
  In/1 -> Transport Delay/1

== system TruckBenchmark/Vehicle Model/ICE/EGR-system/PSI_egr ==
  PI_egr : Inport
  PSI_egr function : Fcn  Expr=1-((1-u)/(1-PI_egropt)-1)^2
  Saturation : Saturate  UpperLimit=1  LowerLimit=PI_egropt
  PSI_egr : Outport
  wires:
  PSI_egr function/1 -> PSI_egr/1
  PI_egr/1 -> Saturation/1
  Saturation/1 -> PSI_egr function/1

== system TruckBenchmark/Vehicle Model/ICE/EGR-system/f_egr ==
  u_egr : Inport
  Constant : Constant  Value=0
  Constant1 : Constant  Value=-c_egr(2)/2/c_egr(1)
  MinMax : MinMax  Function=max  Inputs=2
  MinMax1 : MinMax  Inputs=2
  Polynomial : Polyval  Coefs=c_egr
  f_egr : Outport
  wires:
  Constant1/1 -> MinMax1/2
  MinMax1/1 -> Polynomial/1
  u_egr/1 -> MinMax1/1
  MinMax/1 -> f_egr/1
  Constant/1 -> MinMax/2
  Polynomial/1 -> MinMax/1

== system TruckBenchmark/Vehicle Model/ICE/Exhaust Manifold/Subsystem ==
  p_em : Inport
  T_em : Inport  Port=2
  W_eo : Inport  Port=3
  X_Oe : Inport  Port=4
  Fcn1 : Fcn  Expr=R_e*u[2]/u[1]/V_em*u[3]*(u[4]-u[5])
  Integrator X_Oem : Integrator  LimitOutput=on  UpperSaturationLimit=1  LowerSaturationLimit=0
  Mux1 : Mux  Inputs=5
  X_Oem : Outport
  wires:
  T_em/1 -> Mux1/2
  X_Oe/1 -> Mux1/4
  Integrator X_Oem/1 -> Mux1/5, X_Oem/1
  W_eo/1 -> Mux1/3
  p_em/1 -> Mux1/1
  Fcn1/1 -> Integrator X_Oem/1
  Mux1/1 -> Fcn1/1

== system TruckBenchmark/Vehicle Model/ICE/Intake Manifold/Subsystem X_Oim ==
  p_im : Inport
  T_im : Inport  Port=2
  W_egr : Inport  Port=3
  W_c : Inport  Port=4
  X_Oem : Inport  Port=5
  Fcn1 : Fcn  Expr=R_a*u[2]/u[1]/V_im*(u[3]*(u[5]-u[6])+u[4]*(X_Oc-u[6]))
  Integrator X_Oim : Integrator  InitialCondition=0.2314  LimitOutput=on  UpperSaturationLimit=1  LowerSaturationLimit=0
  Mux1 : Mux  Inputs=6
  X_Oim : Outport
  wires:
  X_Oem/1 -> Mux1/5
  Integrator X_Oim/1 -> Mux1/6, X_Oim/1
  W_c/1 -> Mux1/4
  W_egr/1 -> Mux1/3
  T_im/1 -> Mux1/2
  p_im/1 -> Mux1/1
  Mux1/1 -> Fcn1/1
  Fcn1/1 -> Integrator X_Oim/1

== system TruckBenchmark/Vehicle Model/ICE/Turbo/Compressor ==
  T_bc : Inport
  p_bc : Inport  Port=2
  p_c : Inport  Port=3
  omega_t : Inport  Port=4
  DeltaT_c : Subsystem
  Fcn P_c : Fcn  Expr=u[2]*c_pa*u[1]
  Mux1 : Mux  Inputs=2
  Sub PI_c : Subsystem
  Sub W_c : Subsystem
  Sum : Sum
  W_c : Outport
  T_c : Outport  Port=2
  P_c : Outport  Port=3
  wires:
  Sum/1 -> T_c/1
  Fcn P_c/1 -> [P_c], P_c/1
  Sub W_c/1(W_c) -> W_c/1, [W_c], DeltaT_c/3(W_c), Mux1/2
  omega_t/1 -> Sub W_c/3(omega_t)
  T_bc/1 -> Sub W_c/2(T_bc), DeltaT_c/2(T_bc), Sum/2
  Mux1/1 -> Fcn P_c/1
  DeltaT_c/1(DeltaT_c) -> Sum/1, Mux1/1
  Sub PI_c/1(PI_c) -> DeltaT_c/1(PI_c), Sub W_c/1(PI_c)
  p_bc/1 -> Sub PI_c/2(p_bc), Sub W_c/4(p_bc)
  p_c/1 -> Sub PI_c/1(p_c)

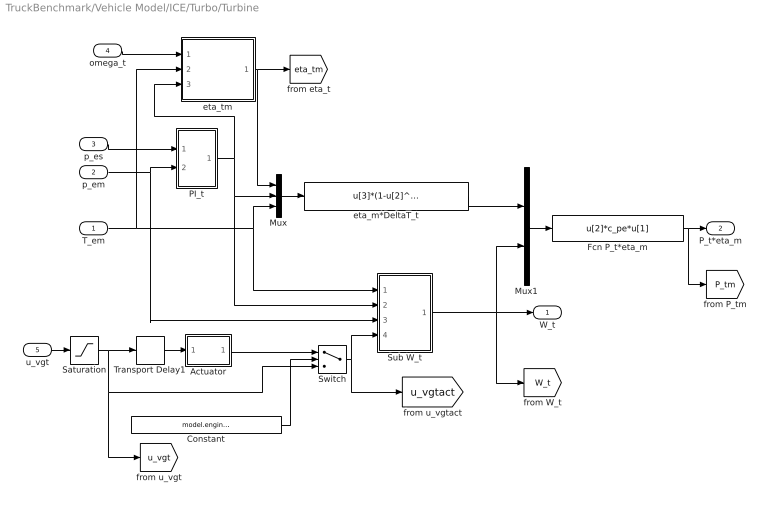
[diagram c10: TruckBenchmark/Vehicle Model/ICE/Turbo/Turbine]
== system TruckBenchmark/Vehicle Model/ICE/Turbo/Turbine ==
  T_em : Inport
  p_em : Inport  Port=2
  p_es : Inport  Port=3
  omega_t : Inport  Port=4
  u_vgt : Inport  Port=5
  Actuator : Subsystem
  Constant : Constant  Value=model.engine.with_vgt_act_model
  Fcn P_t*eta_m : Fcn  Expr=u[2]*c_pe*u[1]
  Mux : Mux  Inputs=3
  Mux1 : Mux  Inputs=2
  PI_t : Subsystem
  Saturation : Saturate  UpperLimit=100  LowerLimit=20
  Sub W_t : Subsystem
  Switch : Switch  Threshold=0.5
  Transport Delay1 : TransportDelay  DelayTime=model.engine.tau_dvgt  InitialOutput=model.engine.uInit_vgt
  eta_m*DeltaT_t : Fcn  Expr=u[3]*(1-u[2]^(1-1/gamma_e))*u[1]
  eta_tm : Subsystem
  W_t : Outport
  P_t*eta_m : Outport  Port=2
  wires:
  Switch/1 -> [u_vgtact], Sub W_t/4(u_vgt)
  Actuator/1(Out) -> Switch/1
  Constant/1 -> Switch/2
  Transport Delay1/1 -> Actuator/1(In)
  u_vgt/1 -> Saturation/1
  eta_tm/1(eta_tm) -> [eta_tm], Mux/1
  Sub W_t/1(W_t) -> [W_t], Mux1/2, W_t/1
  p_es/1 -> PI_t/1(p_es)
  p_em/1 -> Sub W_t/3(p_em), PI_t/2(p_em)
  PI_t/1(PI_t) -> eta_tm/3(PI_t), Sub W_t/2(PI_t), Mux/2
  Mux/1 -> eta_m*DeltaT_t/1
  eta_m*DeltaT_t/1 -> Mux1/1
  Mux1/1 -> Fcn P_t*eta_m/1
  T_em/1 -> eta_tm/2(T_em), Mux/3, Sub W_t/1(T_em)
  omega_t/1 -> eta_tm/1(omega_t)
  Fcn P_t*eta_m/1 -> [P_tm], P_t*eta_m/1
  Saturation/1 -> Switch/3, [u_vgt], Transport Delay1/1

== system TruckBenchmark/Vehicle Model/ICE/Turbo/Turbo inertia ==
  P_t*eta_m : Inport
  P_c : Inport  Port=2
  Divide : Product  Inputs=*/
  Gain : Gain  Gain=1/J_t
  Gain2 : Gain  Gain=30/pi
  Integrator omega_t : Integrator  InitialCondition=omega_t_Init  LimitOutput=on  UpperSaturationLimit=200000*pi/30  LowerSaturationLimit=100*pi/30
  Sum : Sum  Inputs=+-
  omega_t : Outport
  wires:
  Integrator omega_t/1 -> omega_t/1, Gain2/1, Divide/2
  P_c/1 -> Sum/2
  P_t*eta_m/1 -> Sum/1
  Gain2/1 -> [n_t]
  Gain/1 -> Integrator omega_t/1
  Sum/1 -> Divide/1
  Divide/1 -> Gain/1

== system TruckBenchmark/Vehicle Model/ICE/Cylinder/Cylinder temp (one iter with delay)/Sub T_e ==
  PI_e : Inport
  q_in : Inport  Port=2
  T1 : Inport  Port=3
  x_p : Inport  Port=4
  Fcn T_e : Fcn  Expr=eta_sc*u[1]^(1-1/gamma_a)*r_c^(1-gamma_a)*u[4]^(1/gamma_a-1)*(u[2]*((1-x_cv)/c_pa+x_cv/c_va)+u[3]*r_c^(gamma_a-1))
  Mux2 : Mux
  T_e : Outport
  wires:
  Fcn T_e/1 -> T_e/1
  x_p/1 -> Mux2/4
  T1/1 -> Mux2/3
  q_in/1 -> Mux2/2
  PI_e/1 -> Mux2/1
  Mux2/1 -> Fcn T_e/1

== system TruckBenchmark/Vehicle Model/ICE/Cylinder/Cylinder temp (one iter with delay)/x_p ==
  q_in : Inport
  T1 : Inport  Port=2
  Fcn x_p : Fcn  Expr=1+u[1]*x_cv/(c_va*u[2]*r_c^(gamma_a-1))
  Mux1 : Mux  Inputs=2
  x_p : Outport
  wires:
  Fcn x_p/1 -> x_p/1
  T1/1 -> Mux1/2
  q_in/1 -> Mux1/1
  Mux1/1 -> Fcn x_p/1

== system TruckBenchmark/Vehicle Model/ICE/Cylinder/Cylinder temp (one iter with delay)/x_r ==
  x_p : Inport
  T1 : Inport  Port=2
  q_in : Inport  Port=3
  PI_e : Inport  Port=4
  Fcn x_r : Fcn  Expr=u[3]^(1/gamma_a)*u[1]^(-1/gamma_a)/(r_c*u[2])
  Mux4 : Mux  Inputs=2
  Mux5 : Mux  Inputs=3
  x_v : Fcn  Expr=1+u[2]*(1-x_cv)/(c_pa*(u[2]*x_cv/c_va+u[1]*r_c^(gamma_a-1)))
  x_r : Outport
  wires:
  PI_e/1 -> Mux5/3
  q_in/1 -> Mux4/2
  T1/1 -> Mux4/1
  x_p/1 -> Mux5/1
  x_v/1 -> Mux5/2
  Fcn x_r/1 -> x_r/1
  Mux5/1 -> Fcn x_r/1
  Mux4/1 -> x_v/1

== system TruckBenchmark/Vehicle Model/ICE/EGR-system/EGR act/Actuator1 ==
  In : Inport
  Gain : Gain  Gain=1/tau
  Integrator : Integrator  InitialCondition=uInit
  Sum : Sum  Inputs=|+-
  Out : Outport
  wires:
  Gain/1 -> Integrator/1
  Sum/1 -> Gain/1
  Integrator/1 -> Out/1, Sum/2
  In/1 -> Sum/1

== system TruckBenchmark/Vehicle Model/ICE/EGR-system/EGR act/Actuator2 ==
  In : Inport
  Gain : Gain  Gain=1/tau
  Integrator : Integrator  InitialCondition=uInit
  Sum : Sum  Inputs=|+-
  Out : Outport
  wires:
  Gain/1 -> Integrator/1
  Sum/1 -> Gain/1
  Integrator/1 -> Out/1, Sum/2
  In/1 -> Sum/1

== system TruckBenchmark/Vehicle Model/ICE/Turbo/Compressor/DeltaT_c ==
  PI_c : Inport
  T_bc : Inport  Port=2
  W_c : Inport  Port=3
  Fcn DeltaT_c : Fcn  Expr=u[3]*(u[2]^(1-1/gamma_a)-1)/u[1]
  Mux : Mux  Inputs=3
  eta_c : Subsystem
  DeltaT_c : Outport
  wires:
  Fcn DeltaT_c/1 -> DeltaT_c/1
  T_bc/1 -> Mux/3
  PI_c/1 -> Mux/2, eta_c/2(PI_c)
  W_c/1 -> eta_c/1(W_c)
  eta_c/1(eta_c) -> [eta_c], Mux/1
  Mux/1 -> Fcn DeltaT_c/1

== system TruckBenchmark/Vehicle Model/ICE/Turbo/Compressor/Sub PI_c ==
  p_c : Inport
  p_bc : Inport  Port=2
  Constant1 : Constant
  Div PI_c : Product  Inputs=*/
  MinMax1 : MinMax  Function=max  Inputs=2
  PI_c : Outport
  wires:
  MinMax1/1 -> PI_c/1
  p_c/1 -> Div PI_c/1
  p_bc/1 -> Div PI_c/2
  Constant1/1 -> MinMax1/2
  Div PI_c/1 -> MinMax1/1

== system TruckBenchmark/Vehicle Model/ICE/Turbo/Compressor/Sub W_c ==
  PI_c : Inport
  T_bc : Inport  Port=2
  omega_t : Inport  Port=3
  p_bc : Inport  Port=4
  Fcn W_c : Fcn  Expr=u[3]*pi*R_c^3*u[1]*u[4]/(R_a*u[2])
  Mux3 : Mux
  PHI_c : Subsystem
  Saturation : Saturate  UpperLimit=inf  LowerLimit=1e-4
  W_c : Outport
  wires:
  Saturation/1 -> W_c/1  "dm_airInlet"
  Fcn W_c/1 -> Saturation/1
  PI_c/1 -> PHI_c/1(PI_c)
  p_bc/1 -> Mux3/3
  T_bc/1 -> Mux3/2, PHI_c/2(T_bc)
  omega_t/1 -> Mux3/1, PHI_c/3(omega_t)
  PHI_c/1(PHI_c) -> Mux3/4
  Mux3/1 -> Fcn W_c/1

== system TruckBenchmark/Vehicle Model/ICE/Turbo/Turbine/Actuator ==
  In : Inport
  Gain : Gain  Gain=1/tau
  Integrator : Integrator  InitialCondition=uInit
  Sum : Sum  Inputs=|+-
  Out : Outport
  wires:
  Gain/1 -> Integrator/1
  Sum/1 -> Gain/1
  Integrator/1 -> Out/1, Sum/2
  In/1 -> Sum/1

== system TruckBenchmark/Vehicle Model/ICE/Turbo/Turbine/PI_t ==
  p_es : Inport
  p_em : Inport  Port=2
  Constant : Constant  Value=0.9999
  Div PI_t : Product  Inputs=*/
  MinMax : MinMax  Inputs=2
  PI_t : Outport
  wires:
  MinMax/1 -> PI_t/1
  p_es/1 -> Div PI_t/1
  p_em/1 -> Div PI_t/2
  Div PI_t/1 -> MinMax/1
  Constant/1 -> MinMax/2

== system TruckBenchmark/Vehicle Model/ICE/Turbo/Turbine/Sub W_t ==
  T_em : Inport
  PI_t : Inport  Port=2
  p_em : Inport  Port=3
  u_vgt : Inport  Port=4
  Fcn W_t : Fcn  Expr=A_vgtmax*u[3]*sqrt(1-u[2]^K_t)*u[4]/sqrt(u[1]*R_e)
  Mux3 : Mux
  f_vgt : Subsystem
  W_t : Outport
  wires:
  u_vgt/1 -> f_vgt/1(u_vgt)
  Fcn W_t/1 -> W_t/1
  p_em/1 -> Mux3/3
  PI_t/1 -> Mux3/2
  T_em/1 -> Mux3/1
  f_vgt/1(f_vgt) -> Mux3/4
  Mux3/1 -> Fcn W_t/1

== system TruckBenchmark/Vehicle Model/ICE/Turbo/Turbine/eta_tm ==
  omega_t : Inport
  T_em : Inport  Port=2
  PI_t : Inport  Port=3
  BSR : Fcn  Expr=R_t*u[1]/sqrt(2*c_pe*u[2]*(1-u[3]^(1-1/gamma_e)))
  Fcn eta_t : Fcn  Expr=eta_tmmax-u[1]*(u[2]-BSR_opt)^2
  Mux1 : Mux  Inputs=2
  Mux4 : Mux  Inputs=3
  Saturation : Saturate  UpperLimit=2*BSR_opt  LowerLimit=0
  Saturation1 : Saturate  UpperLimit=1  LowerLimit=0.2
  c_m : Subsystem
  eta_tm : Outport
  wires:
  c_m/1(c_m) -> Mux1/1
  Saturation/1 -> [BSR], Mux1/2
  Mux1/1 -> Fcn eta_t/1
  Saturation1/1 -> eta_tm/1
  Fcn eta_t/1 -> Saturation1/1
  PI_t/1 -> Mux4/3
  T_em/1 -> Mux4/2
  omega_t/1 -> c_m/1(omega_t), Mux4/1
  BSR/1 -> Saturation/1
  Mux4/1 -> BSR/1

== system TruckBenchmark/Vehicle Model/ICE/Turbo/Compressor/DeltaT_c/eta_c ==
  W_c : Inport
  PI_c : Inport  Port=2
  Constant2 : Constant  Value=0.2
  Fcn eta_c : Fcn  Expr=eta_cmax-u
  Matrix Gain : Gain  Gain=Q_c  Multiplication=Matrix(K*u)
  MinMax2 : MinMax  Function=max  Inputs=2
  Mux6 : Mux  Inputs=2
  Product : Product  Multiplication=Matrix(*)
  chi1 : Fcn  Expr=u-w_copt
  chi2 : Fcn  Expr=u-pi_copt
  pi_c : Fcn  Expr=(u-1)^c_pi
  transp : Math  Operator=transpose
  eta_c : Outport
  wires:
  W_c/1 -> chi1/1
  MinMax2/1 -> eta_c/1
  PI_c/1 -> pi_c/1
  Constant2/1 -> MinMax2/2
  Fcn eta_c/1 -> MinMax2/1
  Product/1 -> Fcn eta_c/1
  Matrix Gain/1 -> Product/2
  transp/1 -> Product/1
  Mux6/1 -> transp/1, Matrix Gain/1
  chi2/1 -> Mux6/2
  chi1/1 -> Mux6/1
  pi_c/1 -> chi2/1

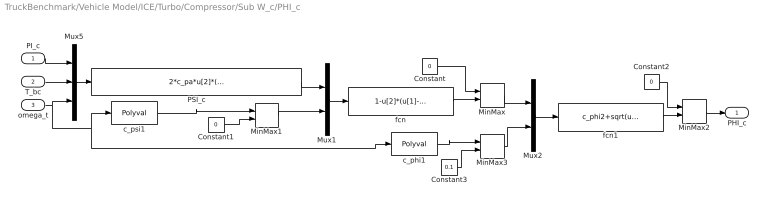
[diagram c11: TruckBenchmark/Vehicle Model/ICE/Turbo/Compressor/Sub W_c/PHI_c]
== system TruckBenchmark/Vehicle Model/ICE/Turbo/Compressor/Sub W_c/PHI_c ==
  PI_c : Inport
  T_bc : Inport  Port=2
  omega_t : Inport  Port=3
  Constant : Constant  Value=0
  Constant1 : Constant  Value=0
  Constant2 : Constant  Value=0
  Constant3 : Constant  Value=0.1
  MinMax{,1..3} (4 alike) : MinMax  Function=max  Inputs=2
  Mux1 : Mux  Inputs=2
  Mux2 : Mux  Inputs=2
  Mux5 : Mux  Inputs=3
  PSI_c : Fcn  Expr=2*c_pa*u[2]*(u[1]^(1-1/gamma_a)-1)/(R_c^2*u[3]^2)
  c_phi1 : Polyval  Coefs=c_wphiVec
  c_psi1 : Polyval  Coefs=c_wpsiVec
  fcn : Fcn  Expr=1-u[2]*(u[1]-c_psi2)^2
  fcn1 : Fcn  Expr=c_phi2+sqrt(u[1]/u[2])
  PHI_c : Outport
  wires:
  Constant3/1 -> MinMax3/2
  MinMax3/1 -> Mux2/2
  c_phi1/1 -> MinMax3/1
  MinMax2/1 -> PHI_c/1
  fcn1/1 -> MinMax2/2
  Constant2/1 -> MinMax2/1
  Mux2/1 -> fcn1/1
  MinMax/1 -> Mux2/1
  fcn/1 -> MinMax/2
  Constant/1 -> MinMax/1
  MinMax1/1 -> Mux1/2
  c_psi1/1 -> MinMax1/1
  Constant1/1 -> MinMax1/2
  Mux1/1 -> fcn/1
  PSI_c/1 -> Mux1/1
  omega_t/1 -> c_phi1/1, c_psi1/1, Mux5/3
  T_bc/1 -> Mux5/2
  PI_c/1 -> Mux5/1
  Mux5/1 -> PSI_c/1

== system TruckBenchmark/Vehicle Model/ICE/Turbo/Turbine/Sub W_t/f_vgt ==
  u_vgt : Inport
  Constant : Constant  Value=0
  Constant1 : Constant  Value=0
  Fcn f_vgt : Fcn  Expr=c_f2+c_f1*sqrt(u)
  Fcn1 : Fcn  Expr=1-((u-c_vgt2)/c_vgt1)^2
  MinMax : MinMax  Function=max  Inputs=2
  MinMax1 : MinMax  Function=max  Inputs=2
  f_vgt : Outport
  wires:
  MinMax1/1 -> f_vgt/1
  Fcn f_vgt/1 -> MinMax1/1
  Constant1/1 -> MinMax1/2
  MinMax/1 -> Fcn f_vgt/1
  Constant/1 -> MinMax/2
  Fcn1/1 -> MinMax/1
  u_vgt/1 -> Fcn1/1

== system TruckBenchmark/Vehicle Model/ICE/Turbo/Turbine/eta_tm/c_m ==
  omega_t : Inport
  Constant : Constant  Value=c_mVec(2)
  MinMax : MinMax  Function=max  Inputs=2
  Switch PSI : Switch  Threshold=w_tlin
  c_m linear : Fcn  Expr=c_mlin*(u-c_mVec(2))/(w_tlin-c_mVec(2))
  c_m power : Fcn  Expr=c_mVec(1)*(u-c_mVec(2))^c_mVec(3)
  c_m : Outport
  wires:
  Switch PSI/1 -> c_m/1
  c_m linear/1 -> Switch PSI/3
  c_m power/1 -> Switch PSI/1
  omega_t/1 -> MinMax/2
  Constant/1 -> MinMax/1
  MinMax/1 -> c_m linear/1, Switch PSI/2, c_m power/1

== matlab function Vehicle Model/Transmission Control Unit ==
function [clutch,gear_out]  = TCU(gear_ref,time)
%#codegen
% Transmission control unit
persistent previous_gear incoming_gear last_state
persistent state t_start last_call
t_declutch=0.5;
t_speed_sync=1.0;
t_onclutch=0.5;


% run initialization
if isempty(state)
  % Initial state
  state=0;
  % Need to set varibles (some to dummy) so that codegen gets to know the size of the
  % persistent variables
  previous_gear=4;
  incoming_gear=4;
  t_start=0;
  previous_gear=gear_ref;
  last_call=time;
  last_state=state;
end
  
% Check if Simulink is restarting with smaller step reduction
if time < last_call,
  if state > 0,
    % disp(['Time reversed during gearchange']);
    if time - t_start < t_declutch,
      state=1;
    elseif time - t_start < t_declutch+t_speed_sync,
      state=2;
    elseif time - t_start < t_declutch+t_speed_sync+t_onclutch
      % backing state_machine
      state=3;
    else
      state=0;
    end
  end
end

last_call=time;
last_state=state;

% Run the state machine
switch state,
  case 0, % 'normal'
    if (gear_ref~=previous_gear)
      t_start=time;
      incoming_gear=gear_ref;
      state=1;
    end
    clutch=1;
    gear_out=previous_gear;
  case 1, % 'ramp_down',
    if ((time-t_start)>t_declutch)
      state=2;
      clutch=0;
    else
      clutch=1-(time-t_start)/t_declutch;
    end    
    gear_out=previous_gear;
  case 2, % 'change_gear',
    if (time>(t_start+t_declutch+t_speed_sync))
      state=3; % 'ramp_up';
      clutch=(time-(t_start+t_declutch+t_speed_sync))/t_onclutch;
    else
      clutch=0;
    end
    gear_out=incoming_gear;
  case 3, % 'ramp_up',
    if (time>(t_start+t_declutch+t_speed_sync+t_onclutch))
      state=0; %'normal';
      clutch=1;
    else
      clutch=(time-(t_start+t_declutch+t_speed_sync))/t_onclutch;
    end
    gear_out=incoming_gear;
    previous_gear=incoming_gear;
  otherwise
    error('Unknown state');
end

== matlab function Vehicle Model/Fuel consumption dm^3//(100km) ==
function fuelConsumption = fcn(m_fuelTot,x_distance)
%#codegen
rho_fuel = 0.8;                               % kg/m^2
if x_distance > 1000
    fuelConsumption = m_fuelTot / (rho_fuel * x_distance / 100000 );   % dm^3/(100km)
else
    fuelConsumption = nan;
end
